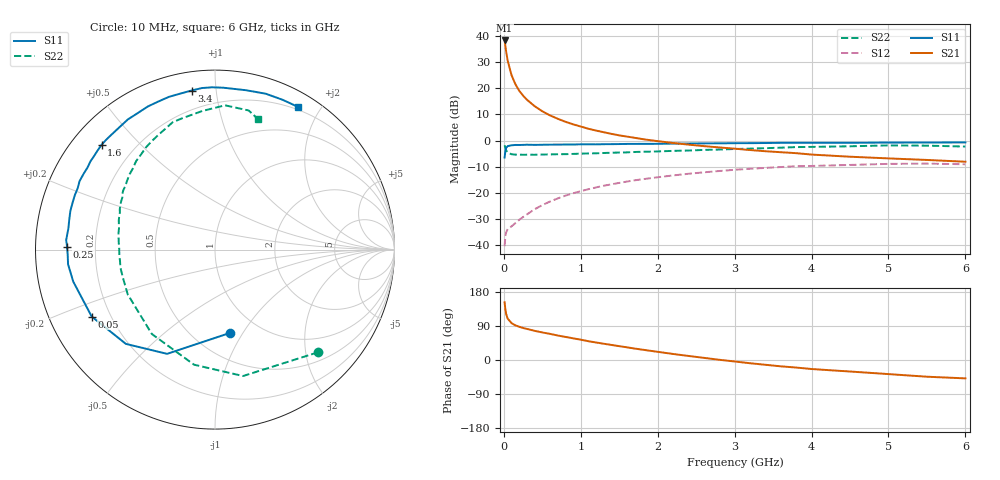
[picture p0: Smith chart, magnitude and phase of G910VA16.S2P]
! SIEMENS Small Signal Semiconductors
! BFG235
! Si NPN RF Bipolar Junction Transistor in SOT223
! VCE = 10 V  IC = 160 mA
! Common Emitter S-Parameters:  July  1994
# GHz  S  MA  R  50
!  f  S11  S21  S12  S22
! GHz  MAG  ANG  MAG  ANG  MAG  ANG  MAG  ANG
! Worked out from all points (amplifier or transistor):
!   40 points, 10 MHz to 6 GHz, reference 50 ohm
!   highest |S21| = 38.4 dB at 10 MHz (marker M1)
!   |S21| within 3 dB of that: start of sweep to 24.19 MHz
!   unconditionally stable (mu >= 1): 454.7 MHz to 1.493 GHz
!   at 200 MHz: K = 0.80, MSG = 24.8 dB, |S12| = -30.4 dB
!   at 1.5 GHz: K = 1.00, MSG = 9.1 dB, |S12| = -16.3 dB
!   at 6 GHz: K = 0.89, MSG = 0.5 dB, |S12| = -9.1 dB
!   S11 on the Smith chart (normalised r, x): 10 MHz: 0.74, -0.88; 50 MHz: 0.13, -0.25; 250 MHz: 0.10, +0.01; 1.6 GHz: 0.09, +0.39; 3.4 GHz: 0.10, +0.86; 6 GHz: 0.17, +1.73
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0.01  0.4714 -79.6  83.16 152.3  0.0094 63.0  0.8104 -44.9
0.02  0.6393 -114.7  65.15 133.3  0.0146 47.5  0.7215 -77.5
0.03  0.7229 -133.4  51.16 121.5  0.0172 40.8  0.6518 -100.3
0.05  0.7818 -151.5  34.01 109.2  0.02 33.9  0.5873 -126.8
0.1  0.8097 -167.3  17.93 97.3  0.0226 36.5  0.5465 -152.8
0.15  0.8227 -174.3  12.05 91.4  0.026 42.7  0.5363 -163.5
0.2  0.8212 -178.0  9.014 87.7  0.0301 46.9  0.5363 -169.3
0.25  0.8242 178.9  7.259 84.5  0.0341 51.3  0.533 -173.1
0.3  0.831 176.3  6.06 82.0  0.0382 54.3  0.534 -176.4
0.4  0.8253 171.9  4.56 77.0  0.048 57.7  0.5338 179.3
0.5  0.8294 168.1  3.64 72.7  0.0577 59.4  0.5376 175.9
0.6  0.8341 165.0  3.037 69.0  0.0675 59.9  0.5416 172.8
0.7  0.8357 161.4  2.618 64.6  0.0775 59.9  0.5457 170.1
0.9  0.838 155.9  2.046 57.2  0.0972 58.0  0.5533 165.4
1.1  0.8451 149.6  1.68 49.5  0.1164 55.6  0.5652 160.8
1.6  0.8603 137.3  1.191 33.5  0.163 47.5  0.5921 150.7
2.2  0.8727 123.8  0.897 15.9  0.214 36.7  0.6333 139.1
3.2  0.8904 102.6  0.657 -8.5  0.287 17.4  0.699 120.4
3.4  0.8959 98.4  0.623 -12.6  0.2984 13.5  0.7134 116.1
4.5  0.9046 79.0  0.489 -30.4  0.34 -7.4  0.7753 95.3
5.5  0.9157 65.7  0.424 -44.1  0.3607 -25.8  0.7975 76.4
6  0.9199 59.7  0.392 -48.5  0.3504 -32.6  0.7656 71.7
